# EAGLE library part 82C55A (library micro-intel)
MICROCOMPUTER/PERIPHERAL DEVICE
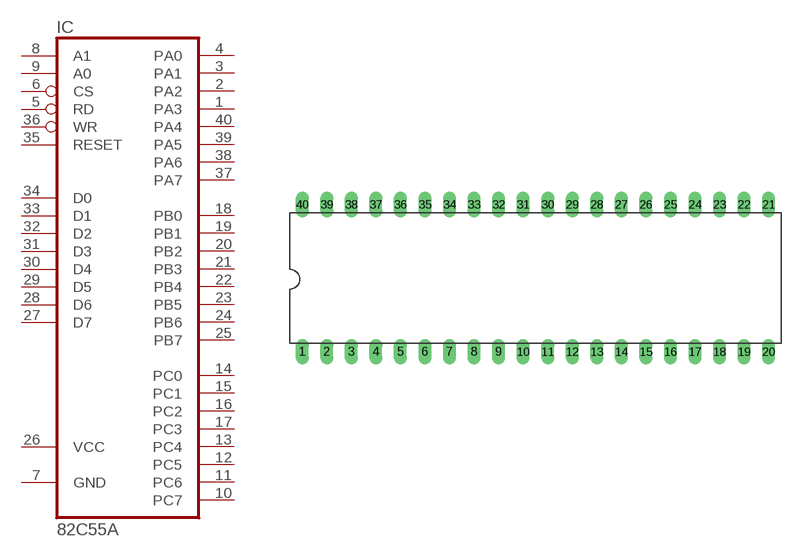
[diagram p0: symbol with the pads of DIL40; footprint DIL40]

Designator prefix IC

## 82C55A (MF: INTERSIL; MPN: IP82C55AZ; OC_FARNELL: 1562050; OC_NEWARK: 79K6939)  [DIL40]
1  PA3
2  PA2
3  PA1
4  PA0
5  RD  in
6  CS  in
7  GND  pwr
8  A1  in
9  A0  in
10  PC7
11  PC6
12  PC5
13  PC4
14  PC0
15  PC1
16  PC2
17  PC3
18  PB0
19  PB1
20  PB2
21  PB3
22  PB4
23  PB5
24  PB6
25  PB7
26  VCC  pwr
27  D7
28  D6
29  D5
30  D4
31  D3
32  D2
33  D1
34  D0
35  RESET  in
36  WR  in
37  PA7
38  PA6
39  PA5
40  PA4

## Footprint DIL40 (pad centres in mm)
Dual In Line Package
drill 0.813 long: 1 -24.13,-7.62; 2 -21.59,-7.62; 3 -19.05,-7.62; 4 -16.51,-7.62; 5 -13.97,-7.62; 6 -11.43,-7.62; 7 -8.89,-7.62; 8 -6.35,-7.62; 9 -3.81,-7.62; 10 -1.27,-7.62; 11 1.27,-7.62; 12 3.81,-7.62; 13 6.35,-7.62; 14 8.89,-7.62; 15 11.43,-7.62; 16 13.97,-7.62; 17 16.51,-7.62; 18 19.05,-7.62; 19 21.59,-7.62; 20 24.13,-7.62; 21 24.13,7.62; 22 21.59,7.62; 23 19.05,7.62; 24 16.51,7.62; 25 13.97,7.62; 26 11.43,7.62; 27 8.89,7.62; 28 6.35,7.62; 29 3.81,7.62; 30 1.27,7.62; 31 -1.27,7.62; 32 -3.81,7.62; 33 -6.35,7.62; 34 -8.89,7.62; 35 -11.43,7.62; 36 -13.97,7.62; 37 -16.51,7.62; 38 -19.05,7.62; 39 -21.59,7.62; 40 -24.13,7.62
